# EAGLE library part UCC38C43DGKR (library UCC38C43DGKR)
BiCMOS Low-Power Current Mode PWM Controller Source: Datasheet
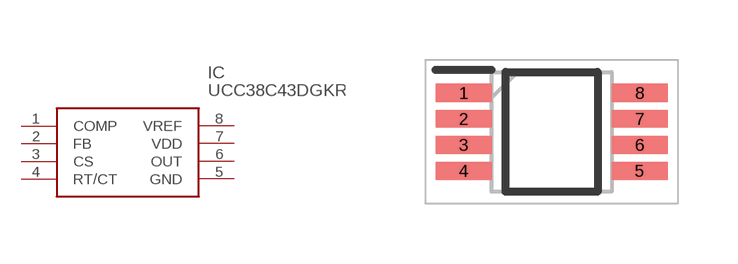
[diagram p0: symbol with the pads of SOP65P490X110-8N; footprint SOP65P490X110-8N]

Designator prefix IC

## UCC38C43DGKR (Description: BiCMOS Low-Power Current Mode PWM Controller; Height: 1.1mm; Manufacturer_Name: Texas Instruments; Manufacturer_Part_Number: UCC38C43DGKR; Mouser_Part_Number: 595-UCC38C43DGKR; Mouser_Price-Stock: https://www.mouser.co.uk/ProductDetail/Texas-Instruments/UCC38C43DGKR?qs=zqbRmZ%252BfZD%252BXDziCZUmxYw%3D%3D)  [SOP65P490X110-8N]
1  COMP
2  FB
3  CS
4  RT/CT
5  GND
6  OUT
7  VDD
8  VREF

## Footprint SOP65P490X110-8N (pad centres in mm)
DGK (S-PDSO-G8)
smd 1.4 x 0.45: 1 -2.2,0.975; 2 -2.2,0.325; 3 -2.2,-0.325; 4 -2.2,-0.975; 5 2.2,-0.975; 6 2.2,-0.325; 7 2.2,0.325; 8 2.2,0.975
